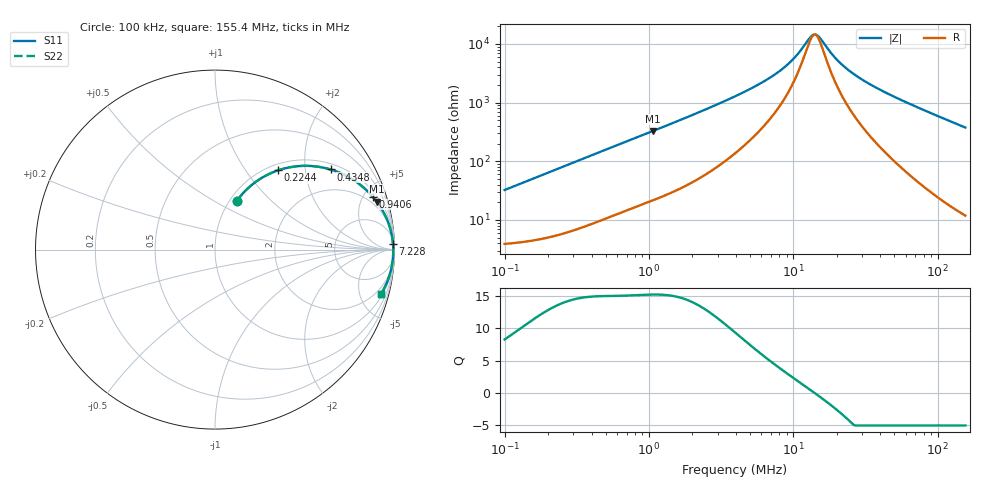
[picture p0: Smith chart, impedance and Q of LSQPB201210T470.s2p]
! LSQPB201210T470  S-PARAMETER MODEL  ( General Type )
! Model Generated by TAIYO YUDEN Corporation (http://www.ty-top.com)
! Version 2.0
! TAIYO YUDEN Control No. 100810NF18SB-HKC
! Copyright(c) 2007 TAIYO YUDEN CO.,LTD. All Rights Reserved.
! Product Description (link to TY-COMPAS)
! https://ds.yuden.co.jp/TYCOMPAS/or/detail?pn=LSQPB201210T470M&u=M
! Products Name : Inductors
! Characteristics :
!  Inductance : 47 uH , SRF(min) : 7.0 MHz , DC Resistance(max) : 4.55 Ohm
!  Rated Current : Saturation :125 mA , Temp Rise : 160 mA (40 degC)
!  Case Size : 2.0 x 1.25 / 0.079 x 0.049 [mm/inch] , Thickness : 1.0 / 0.04 [mm/inch]
!  (Conditions: Temperature = 25 degC , DC Bias Current/Voltage = 0A / 0V)
! External Node Assignments :
!  1  o---GGG---o  2
! GND o---------o GND
! Frequency Range : 0.1MHz  -  155.401204MHz  [ 402 STEP ]
# MHz S RI R 50
! Freq[MHz].  S11 Real  S11 Imag  S21 Real  S21 Imag  S12 Real  S12 Imag  S22 Real  S22 Imag
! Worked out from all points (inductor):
!   401 points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, 100 kHz to 155.4 MHz, reference 50 ohm
!   read as one part in series: L = 51.1 uH near 103.7 kHz
!   highest Q = 15.2 at 1.07 MHz (marker M1), where L = 48.9 uH
!   self-resonance near 14 MHz
!   S11 on the Smith chart (normalised r, x): 100 kHz: 1.08, +0.64; 224.4 kHz: 1.11, +1.43; 434.8 kHz: 1.18, +2.74; 940.6 kHz: 1.38, +5.79; 7.228 MHz: 13, +56; 155.4 MHz: 1.24, -7.51
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0.1  0.1215 0.2716  0.8785 -0.2716  0.8785 -0.2716  0.1215 0.2716
0.149806  0.2093 0.3639  0.7907 -0.3639  0.7907 -0.3639  0.2093 0.3639
0.224419  0.3512 0.4414  0.6488 -0.4414  0.6488 -0.4414  0.3512 0.4414
0.342427  0.5395 0.4655  0.4605 -0.4655  0.4605 -0.4655  0.5395 0.4655
0.434801  0.6443 0.4463  0.3557 -0.4463  0.3557 -0.4463  0.6443 0.4463
0.639502  0.7842 0.3794  0.2158 -0.3794  0.2158 -0.3794  0.7842 0.3794
0.940575  0.8785 0.2953  0.1215 -0.2953  0.1215 -0.2953  0.8785 0.2953
1.069656  0.9009 0.2677  0.0991 -0.2677  0.0991 -0.2677  0.9009 0.2677
1.172566  0.9144 0.2487  0.0856 -0.2487  0.0856 -0.2487  0.9144 0.2487
2.110832  0.9668 0.1465  0.0332 -0.1465  0.0332 -0.1465  0.9668 0.1465
3.942096  0.9859 0.076  0.0141 -0.076  0.0141 -0.076  0.9859 0.076
7.228067  0.9915 0.0334  0.00846 -0.0334  0.00846 -0.0334  0.9915 0.0334
9.877772  0.9926 0.0169  0.00736 -0.0169  0.00736 -0.0169  0.9926 0.0169
13.49882  0.9931 0.00191  0.00686 -0.00191  0.00686 -0.00191  0.9931 0.00191
14.26368  0.9932 -0.000683  0.00682 0.000683  0.00682 0.000683  0.9932 -0.000683
15.07189  0.9932 -0.00328  0.00679 0.00328  0.00679 0.00328  0.9932 -0.00328
19.49254  0.9931 -0.0157  0.00686 0.0157  0.00686 0.0157  0.9931 -0.0157
24.75089  0.9927 -0.0283  0.00727 0.0283  0.00727 0.0283  0.9927 -0.0283
32.60396  0.9916 -0.0448  0.00836 0.0448  0.00836 0.0448  0.9916 -0.0448
46.22367  0.9887 -0.0709  0.0113 0.0709  0.0113 0.0709  0.9887 -0.0709
86.32529  0.9732 -0.1401  0.0268 0.1401  0.0268 0.1401  0.9732 -0.1401
155.4012  0.9271 -0.2446  0.0729 0.2446  0.0729 0.2446  0.9271 -0.2446
